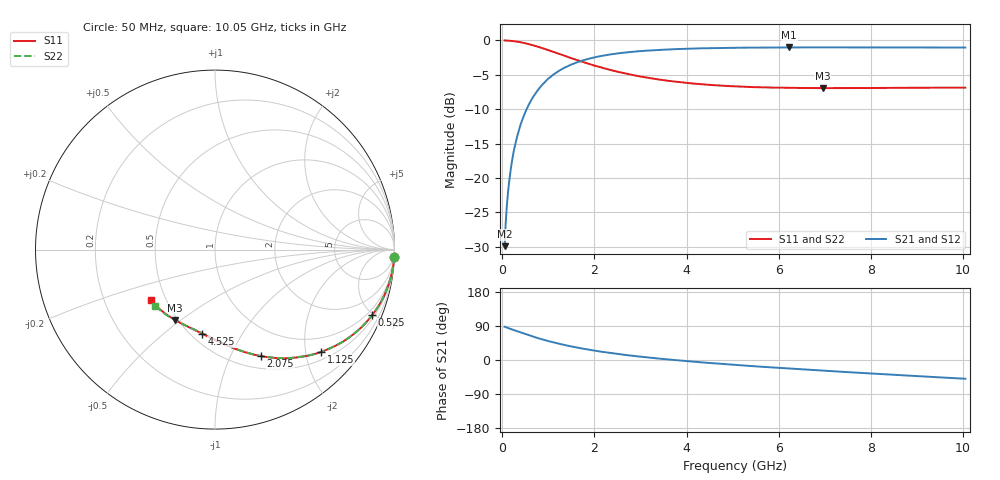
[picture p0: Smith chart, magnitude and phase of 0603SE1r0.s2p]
! fin_1r9! AVX Thin Film Operation		Date: August 2001
! Description: Accu-P® Series, Thin Film, SMD, RF Capacitor
! Part Number: 06035J1R0ABT
! 50 MHz  -  10.05 GHz
! Serial Measurements
# mhz S db R 50
!	S11		S21		S12		S22
!	dB	Phase	dB	Phase	dB	Phase	dB	Phase
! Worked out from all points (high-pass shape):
!   401 points, 50 MHz to 10.05 GHz, reference 50 ohm
!   highest |S21| = -1.01 dB at 6.225 GHz (marker M1); lowest = -29.9 dB at 50 MHz (marker M2)
!   |S21| within 3 dB of the highest: 1.337 GHz to end of sweep
!   lowest |S11| = -6.9 dB at 6.95 GHz (marker M3), VSWR 2.64, Z = 24.2 - j23.8 ohm
!   |S11| at or under -10 dB: nowhere
!   |S22| runs from -6.9 to 0.0 dB; largest |S21 - S12| = 0
!   S11 on the Smith chart (normalised r, x): 50 MHz: 1, -51; 525 MHz: 0.67, -4.89; 1.125 GHz: 0.66, -2.32; 2.075 GHz: 0.64, -1.31; 4.525 GHz: 0.57, -0.69; 10.05 GHz: 0.41, -0.29
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50  -0.00 -2.2  -29.90 87.8  -29.90 87.8  -0.00 -2.2
75  -0.01 -3.3  -26.41 86.6  -26.41 86.6  -0.01 -3.3
125  -0.03 -5.6  -21.99 84.4  -21.99 84.4  -0.03 -5.6
150  -0.04 -6.7  -20.47 83.3  -20.47 83.3  -0.04 -6.7
225  -0.09 -10.0  -16.96 80.1  -16.96 80.1  -0.09 -10.0
275  -0.13 -12.2  -15.28 77.8  -15.28 77.8  -0.13 -12.2
350  -0.21 -15.4  -13.29 74.6  -13.29 74.6  -0.21 -15.4
525  -0.46 -22.7  -10.02 67.3  -10.02 67.3  -0.46 -22.7
800  -0.97 -33.1  -6.98 56.9  -6.98 56.9  -0.97 -33.1
1125  -1.71 -43.9  -4.90 46.1  -4.90 46.1  -1.71 -43.9
1375  -2.30 -51.1  -3.88 38.9  -3.88 38.9  -2.30 -51.1
1725  -3.08 -59.6  -2.95 30.4  -2.95 30.4  -3.08 -59.5
2075  -3.79 -66.7  -2.35 23.3  -2.35 23.3  -3.79 -66.5
2625  -4.74 -76.1  -1.79 14.0  -1.79 14.0  -4.73 -75.8
3400  -5.68 -86.4  -1.38 3.8  -1.38 3.8  -5.67 -85.9
4525  -6.47 -98.5  -1.12 -8.1  -1.12 -8.1  -6.46 -97.5
5050  -6.68 -103.6  -1.06 -12.9  -1.06 -12.9  -6.67 -102.0
6225  -6.89 -113.2  -1.01 -22.6  -1.01 -22.6  -6.88 -111.2
6725  -6.92 -117.0  -1.01 -26.5  -1.01 -26.5  -6.90 -114.9
6950  -6.93 -119.5  -1.01 -28.1  -1.01 -28.1  -6.91 -116.5
8400  -6.90 -130.2  -1.02 -38.4  -1.02 -38.4  -6.87 -126.2
10050  -6.86 -141.8  -1.03 -49.5  -1.03 -49.5  -6.83 -136.8
